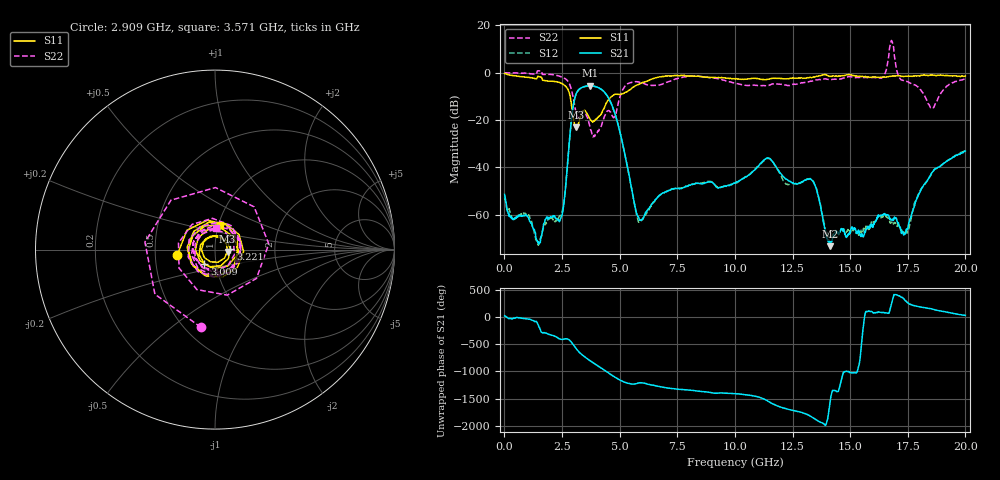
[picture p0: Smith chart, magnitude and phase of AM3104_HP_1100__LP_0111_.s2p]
!Created with skrf (http://scikit-rf.org).
# Hz S RI R 50.0
!freq ReS11 ImS11 ReS21 ImS21 ReS12 ImS12 ReS22 ImS22
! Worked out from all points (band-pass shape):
!   1601 points, 10 MHz to 20 GHz, reference 50 ohm
!   highest |S21| = -5.51 dB at 3.708 GHz (marker M1); lowest = -73.2 dB at 14.14 GHz (marker M2)
!   |S21| within 3 dB of the highest: 3.134 GHz to 4.364 GHz (1.229 GHz wide, 32.8 % of centre)
!   lowest |S11| = -23.0 dB at 3.096 GHz (marker M3), VSWR 1.15, Z = 57.5 - j1.26 ohm
!   |S11| at or under -10 dB: 2.851 GHz to 4.662 GHz (1.811 GHz wide, 48.2 % of centre)
!   |S22| runs from -27.1 to 13.6 dB; largest |S21 - S12| = 0.036
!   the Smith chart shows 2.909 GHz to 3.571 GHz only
!   S11 on the Smith chart (normalised r, x): 2.909 GHz: 0.65, -0.04; 3.009 GHz: 0.88, -0.14; 3.221 GHz: 1.19, +0.01; 3.571 GHz: 1.01, +0.29
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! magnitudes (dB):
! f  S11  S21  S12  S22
! 10 MHz  -0.4  -51.3  -52.7  -0.1
! 1.447 GHz  -1.6  -71.5  -72.2  0.8
! 2.409 GHz  -4.2  -62.5  -60.6  -1.6
! 2.909 GHz  -13.5  -19.9  -20.0  -7.1
! 3.009 GHz  -20.0  -12.8  -12.9  -11.6
! 3.096 GHz  -23.0  -9.4  -9.4  -16.4
! 3.221 GHz  -21.3  -7.2  -7.3  -19.1
! 3.346 GHz  -17.6  -6.3  -6.4  -16.9
! 3.571 GHz  -17.0  -5.6  -5.7  -18.3
! 3.708 GHz  -19.5  -5.5  -5.6  -22.7
! 4.733 GHz  -9.5  -15.5  -15.5  -19.0
! 5.82 GHz  -5.0  -60.9  -63.1  -3.9
! 6.682 GHz  -1.9  -52.3  -52.2  -5.3
! 10.01 GHz  -2.7  -46.6  -46.8  -4.5
! 11.44 GHz  -2.8  -36.0  -36.1  -5.5
! 13.34 GHz  -2.1  -45.3  -45.4  -3.6
! 14.14 GHz  -1.6  -73.2  -68.9  -3.0
! 16.36 GHz  -1.9  -60.1  -60.6  -2.3
! 16.68 GHz  -1.6  -60.2  -62.4  7.1
! 17.4 GHz  -1.5  -67.8  -66.8  -3.5
! 18.54 GHz  -1.0  -42.3  -42.4  -14.6
! 20 GHz  -1.4  -33.1  -32.9  -2.7
